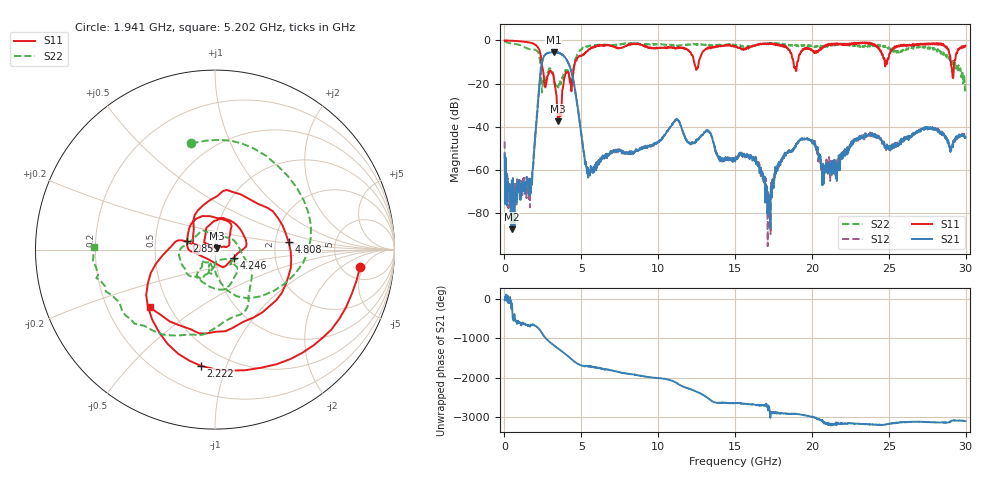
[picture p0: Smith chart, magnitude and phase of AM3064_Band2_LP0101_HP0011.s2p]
# Hz S DB R 50.0
!freq dBS11 angS11 dBS21 angS21 dBS12 angS12 dBS22 angS22
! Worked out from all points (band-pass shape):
!   1600 points, 10 MHz to 29.98 GHz, reference 50 ohm
!   highest |S21| = -5.35 dB at 3.215 GHz (marker M1); lowest = -87.6 dB at 459.8 MHz (marker M2)
!   |S21| within 3 dB of the highest: 2.514 GHz to 3.976 GHz (1.462 GHz wide, 45.1 % of centre)
!   lowest |S11| = -37.5 dB at 3.478 GHz (marker M3), VSWR 1.03, Z = 51 + j0.848 ohm
!   |S11| at or under -10 dB: 2.418 GHz to 4.595 GHz (2.176 GHz wide, 62.1 % of centre); 12.33 GHz to 12.64 GHz (312.1 MHz wide, 2.5 % of centre); 18.8 GHz to 19.05 GHz (253.2 MHz wide, 1.34 % of centre)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
!   |S22| runs from -24.2 to -0.2 dB; largest |S21 - S12| = 0.014
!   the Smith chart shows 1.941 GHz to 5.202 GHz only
!   S11 on the Smith chart (normalised r, x): 1.941 GHz: 7.20, -4.24; 2.222 GHz: 0.36, -0.82; 2.859 GHz: 0.73, +0.07; 4.246 GHz: 1.22, -0.11; 4.808 GHz: 2.37, +0.24; 5.202 GHz: 0.39, -0.33
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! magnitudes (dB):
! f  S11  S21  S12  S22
! 10 MHz  0.0  -52.8  -46.9  -0.2
! 459.8 MHz  -0.2  -87.6  -74.5  -1.4
! 1.659 GHz  -1.0  -67.8  -77.4  -4.1
! 1.941 GHz  -1.8  -50.0  -49.8  -4.3
! 2.222 GHz  -3.7  -25.1  -25.0  -6.1
! 2.859 GHz  -15.8  -5.8  -5.8  -14.2
! 3.215 GHz  -17.7  -5.3  -5.5  -18.3
! 3.478 GHz  -37.5  -5.5  -5.6  -21.4
! 4.246 GHz  -18.9  -11.9  -11.9  -17.9
! 4.808 GHz  -7.7  -33.4  -33.3  -5.6
! 5.015 GHz  -7.3  -44.1  -44.1  -4.3
! 5.202 GHz  -6.3  -53.9  -54.2  -3.4
! 10 GHz  -3.5  -47.2  -47.1  -1.9
! 11.24 GHz  -3.7  -36.6  -36.5  -2.6
! 15 GHz  -2.7  -56.2  -55.0  -2.0
! 16.32 GHz  -2.2  -55.9  -54.5  -2.1
! 17.24 GHz  -1.5  -71.9  -75.2  -1.3
! 18.19 GHz  -2.4  -53.4  -52.8  -1.9
! 19.99 GHz  -4.4  -46.3  -46.6  -2.3
! 20.74 GHz  -3.2  -59.2  -58.9  -2.9
! 25 GHz  -8.0  -49.1  -49.8  -3.2
! 29.98 GHz  -2.5  -45.2  -44.5  -20.2
